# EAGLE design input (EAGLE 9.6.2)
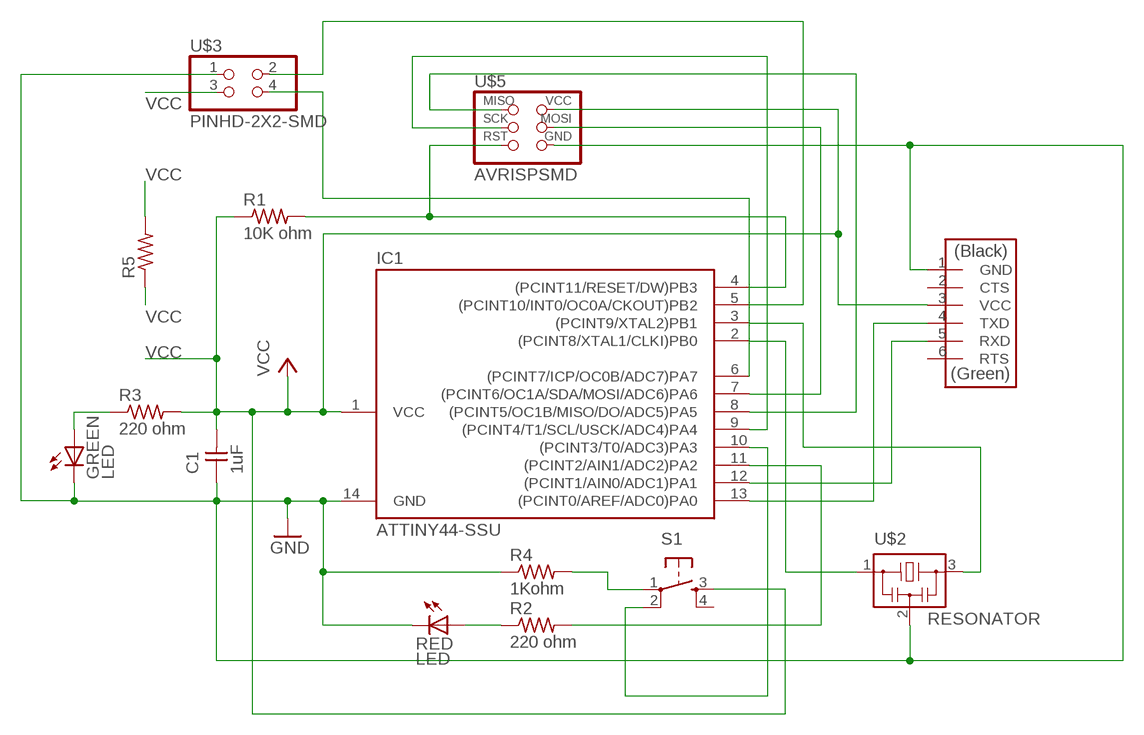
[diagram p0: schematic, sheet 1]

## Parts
C1  1uF  CAP-UNPOLARIZED  [C1206]
GREEN  LED  [LED1206]
IC1  ATTINY44-SSU  [SOIC14]
R1  10K ohm  RES-US1206  [R1206]
R2  220 ohm  RES-US1206  [R1206]
R3  220 ohm  RES-US1206  [R1206]
R4  1Kohm  RES-US1206  [R1206]
R5  RES-US1206  [R1206]
RED  LED  [LED1206]
S1  6MM_SWITCH6MM_SWITCH  [6MM_SWITCH]
U$1  FTDI-SMD-HEADER  [1X06SMD]
U$2  RESONATOR  [EFOBM]
U$3  PINHD-2X2-SMD  [2X02SMD]
U$5  AVRISPSMD  [2X03SMD]

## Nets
GND: C1.1 GREEN.2(C) IC1.14(GND) R4.1 RED.2(C) U$1.1(GND) U$2.2 U$3.1 U$5.6(GND)
N$1: R4.2 S1.1(P)
N$2: IC1.3((PCINT9/XTAL2)PB1) U$2.3
N$3: IC1.7((PCINT6/OC1A/SDA/MOSI/ADC6)PA6) U$5.4(MOSI)
N$4: IC1.4((PCINT11/RESET/DW)PB3) R1.2 U$5.5(RST)
N$5: IC1.2((PCINT8/XTAL1/CLKI)PB0) U$2.1
N$6: IC1.12((PCINT1/AIN0/ADC1)PA1) U$1.5(RXD)
N$7: IC1.13((PCINT0/AREF/ADC0)PA0) U$1.4(TXD)
N$8: IC1.9((PCINT4/T1/SCL/USCK/ADC4)PA4) U$5.3(SCK)
N$9: IC1.11((PCINT2/AIN1/ADC2)PA2) R2.2
N$10: IC1.8((PCINT5/OC1B/MISO/DO/ADC5)PA5) U$5.1(MISO)
N$11: IC1.10((PCINT3/T0/ADC3)PA3) S1.2(P1)
N$12: R2.1 RED.1(A)
N$13: GREEN.1(A) R3.1
N$14: IC1.5((PCINT10/INT0/OC0A/CKOUT)PB2) U$3.2
N$15: IC1.6((PCINT7/ICP/OC0B/ADC7)PA7) U$3.4
VCC: C1.2 IC1.1(VCC) R1.1 R3.2 R5.1 R5.2 S1.3(S) U$1.3(VCC) U$3.3 U$5.2(VCC)
Unconnected: S1.4(S1) U$1.2(CTS) U$1.6(RTS)

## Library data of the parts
C1 = fab:CAP-UNPOLARIZED
GREEN RED = fab:LED: LED
IC1 = fab:ATTINY44
R1-R5 = fab:RES-US: Resistor (US Symbol)
S1 = fab:6MM_SWITCH: OMRON SWITCH
U$1 = fab:FTDI-SMD-HEADER
U$2 = fab:RESONATOR
U$3 = fab:PINHD-2X2-SMD
U$5 = fab:AVRISP

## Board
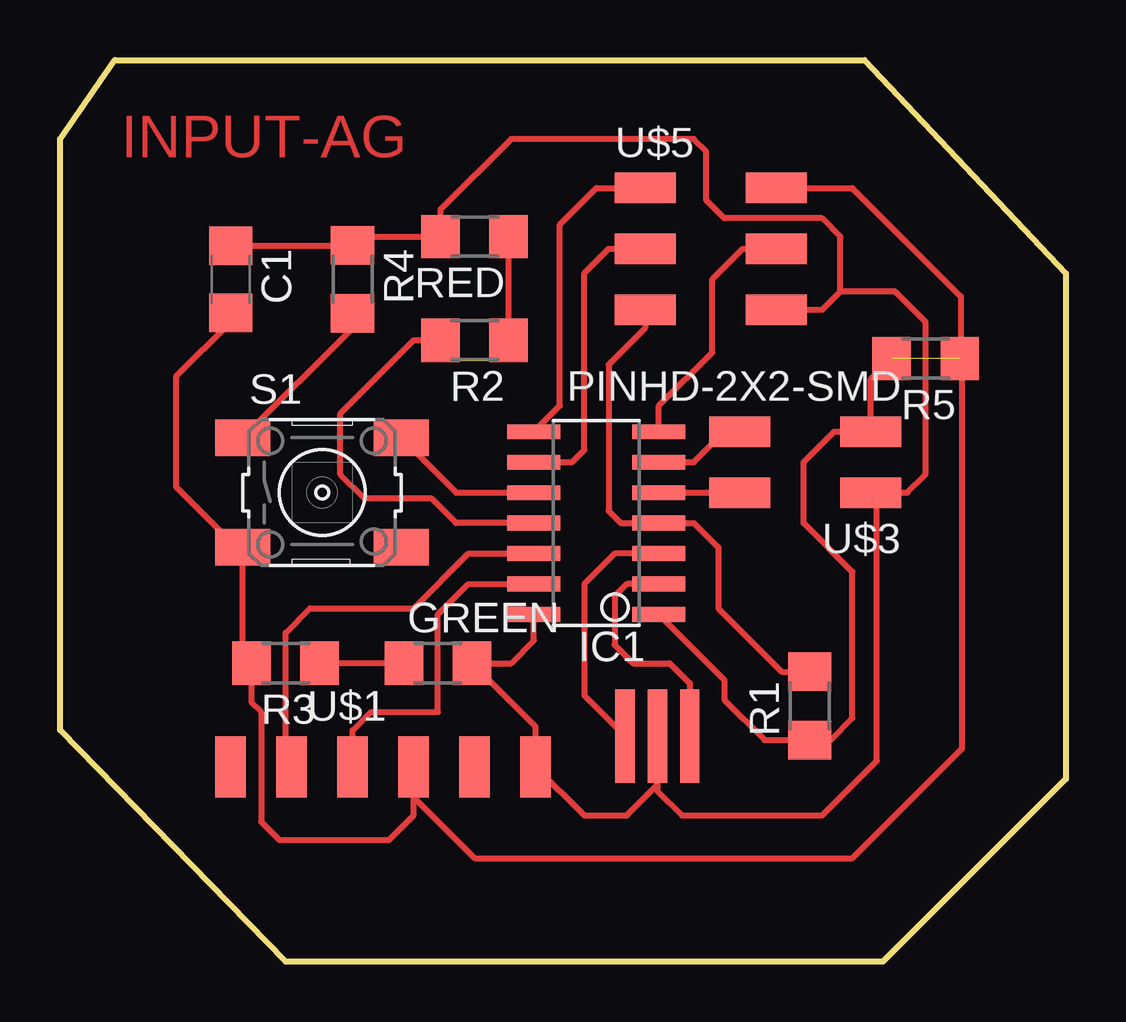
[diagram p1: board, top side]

Size 41.91 x 37.59 mm. Coordinates in mm from the lower left corner, seen from the top.
Outline: 2.29,37.59 33.53,37.59 41.91,28.7 41.91,7.62 34.29,0 9.4,0 0,9.65 0,34.29 2.29,37.59
Copper layers (1*16): Top 0.035mm / dielectric 1.5mm / Bottom 0.035mm
Design rules "default": minimum track width 6mil, minimum drill 0.35mm, track to track 6mil, track to pad 6mil, pad to pad 6mil, via to via 6mil, smd to smd 6mil, copper to edge 40mil, drill to drill 6mil, minimum pad ring 10mil, minimum via ring 8mil, stop-mask expansion 4mil, vias tented up to drill 0mil, thermal gap 10mil

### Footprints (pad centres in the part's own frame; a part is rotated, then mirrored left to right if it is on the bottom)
C1206 = smd 1.6 x 1.8: 1 -1.4,0; 2 1.4,0
LED1206 = smd 1.6 x 1.803: 1 -1.422,0; 2 1.422,0
SOIC14 = smd 0.61 x 2.21: 1 -3.81,-2.603; 2 -2.54,-2.603; 3 -1.27,-2.603; 4 0,-2.603; 5 1.27,-2.603; 6 2.54,-2.603; 7 3.81,-2.603; 8 3.81,2.603; 9 2.54,2.603; 10 1.27,2.603; 11 0,2.603; 12 -1.27,2.603; 13 -2.54,2.603; 14 -3.81,2.603
R1206 = smd 1.6 x 1.803: 1 -1.422,0; 2 1.422,0
6MM_SWITCH = smd 2.286 x 1.524: 1 -3.302,2.286; 2 3.302,2.286; 3 -3.302,-2.286; 4 3.302,-2.286
1X06SMD = smd 2.54 x 1.27: 1 0,6.35; 2 0,3.81; 3 0,1.27; 4 0,-1.27; 5 0,-3.81; 6 0,-6.35
EFOBM = smd 0.8 x 3.9: 1 -1.35,0; 2 0,0; 3 1.35,0
2X02SMD = smd 2.54 x 1.27: 1 -2.54,1.27; 2 2.92,1.27; 3 -2.54,-1.27; 4 2.92,-1.27
2X03SMD = smd 2.54 x 1.27: 1 -2.54,2.54; 2 2.92,2.54; 3 -2.54,0; 4 2.92,0; 5 -2.54,-2.54; 6 2.92,-2.54

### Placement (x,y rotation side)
C1  7.11,28.45 270 top
GREEN  15.75,12.45 0 top
IC1  22.35,18.29 90 top
R1  31.24,10.67 90 top
R2  17.27,25.91 180 top
R3  9.4,12.45 180 top
R4  12.19,28.45 270 top
R5  36.07,25.15 180 top
RED  17.27,30.23 180 top
S1  10.92,19.56 0 top
U$1  13.46,8.13 270 top
U$2  24.89,9.4 180 top
U$3  31.24,20.83 180 top
U$5  26.92,29.72 0 top

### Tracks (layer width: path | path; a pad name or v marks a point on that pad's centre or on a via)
GND
  Top 0.254: IC1.14 19.75,13.4 18.8,12.45 GREEN.2 19.81,9.8 U$1.1 21.84,6.1 23.62,6.1 24.89,7.37 U$2.2 24.89,7.11 25.91,6.1 31.75,6.1 34.04,8.38 34.04,19.3 U$3.1 35.31,19.56 36.07,20.32 36.07,26.67 34.8,27.94 32.51,27.94 | C1.1 12.17,29.85 R4.1 12.55,30.23 RED.2 15.85,31.34 18.8,34.29 26.42,34.29 26.92,33.78 26.92,31.75 27.69,30.99 31.75,30.99 32.51,30.23 32.51,27.94 | U$5.6 31.75,27.18 32.51,27.94
N$1
  Top 0.254: S1.1 12.19,26.42 R4.2
N$2
  Top 0.254: IC1.3 23.11,17.02 21.84,15.75 21.84,11.1 U$2.3
N$3
  Top 0.254: IC1.7 24.96,23.18 27.18,25.4 27.18,28.45 28.45,29.72 U$5.4
N$4
  Top 0.254: R1.2 30.07,12.09 27.43,14.73 27.43,17.27 26.42,18.29 IC1.4 23.37,18.29 22.86,18.8 22.86,24.89 24.38,26.42 U$5.5
N$5
  Top 0.254: IC1.2 23.62,15.75 23.11,15.24 23.11,13.21 23.88,12.45 25.4,12.45 26.24,11.6 U$2.1
N$6
  Top 0.254: U$1.5 9.4,8.38 9.4,13.72 10.41,14.73 14.73,14.73 17.02,17.02 IC1.12
N$7
  Top 0.254: U$1.4 12.19,9.65 12.95,10.41 15.75,10.41 15.75,14.48 17.02,15.75 IC1.13
N$8
  Top 0.254: IC1.9 21.34,20.83 21.84,21.34 21.84,28.7 22.86,29.72 U$5.3
N$9
  Top 0.254: IC1.11 16.51,18.29 15.49,19.3 12.7,19.3 11.68,20.32 11.68,22.86 14.73,25.91 R2.2
N$10
  Top 0.254: IC1.8 20.83,23.18 20.83,30.73 22.35,32.26 U$5.1
N$11
  Top 0.254: S1.2 16.51,19.56 IC1.10
N$12
  Top 0.254: R2.1 RED.1
N$13
  Top 0.254: GREEN.1 R3.1
N$14
  Top 0.254: IC1.5 U$3.2
N$15
  Top 0.254: IC1.6 26.42,20.83 27.69,22.1 U$3.4
VCC  (1 unrouted)
  Top 0.254: IC1.1 27.69,11.75 27.69,10.92 29.36,9.25 R1.1 32.11,9.25 33.02,10.16 33.02,16.26 30.99,18.29 30.99,20.83 32.26,22.1 U$3.3 33.78,24.28 R5.2 | 7.62,17.02 7.62,12.8 R3.2 7.98,10.82 8.38,10.41 8.38,5.84 9.14,5.08 13.72,5.08 14.73,6.1 U$1.3 14.73,6.86 17.27,4.32 33.02,4.32 37.59,8.89 37.59,24.79 37.54,24.84 37.54,25.09 | 7.62,17.02 S1.3 | C1.2 7.11,26.67 4.83,24.38 4.83,19.81 7.62,17.02 | U$5.2 33.02,32.26 37.54,27.74 37.54,25.09 | 37.54,25.09 R5.1

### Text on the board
Top: INPUT-AG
